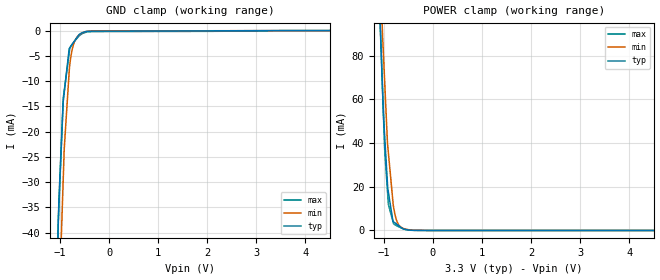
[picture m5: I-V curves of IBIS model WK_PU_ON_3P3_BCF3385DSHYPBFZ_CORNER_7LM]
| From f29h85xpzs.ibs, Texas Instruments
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|RECEIVER_MODE_3P3; RECEIVER_MODE
|   Model Cell WK_PU_ON_3P3_BCF3385DSHYPBFZ_CORNER_7LM
|WK_PU_ON_3P3_BCF3385DSHYPBFZ_CORNER_7LM
[Model]   WK_PU_ON_3P3_BCF3385DSHYPBFZ_CORNER_7LM
Model_type   Input
Polarity   Non-Inverting
Vinl = 0.8
Vinh = 2
|   typ   min   max
C_comp   0.44pF   0.4pF   0.46pF
[Model Spec]
Vinl   0.8   0.8   0.8
Vinh   2   2   2
[Temperature Range]   25   155   -40
[Voltage Range]   3.3   2.8   3.63
| Nom Voltages:
|   VDD=1.23, VDDS=3.3, VSS=0
| Min Voltages:
|   VDD=1.08, VDDS=2.8, VSS=0
| Max Voltages:
|   VDD=1.32, VDDS=3.63, VSS=0
[Power Clamp Reference]   3.3   2.8   3.63
[GND Clamp Reference]   0   0   0
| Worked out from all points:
|   GND clamp passes 1 mA (typ) near -0.63 V on its own axis
|   POWER clamp passes 1 mA (typ) near -0.63 V on its own axis
[GND Clamp]
|   Voltage   I(typ)   I(min)   I(max)
-3.3V     -1.475A    -1.211A    -2.162A
-1.048V   -42.98mA   -65.6mA    -41.49mA
-1.04V    -39.54mA   -62.41mA   -38.5mA
-1.024V   -33.55mA   -55.94mA   -34.71mA
-1.014V   -31.3mA    -52.41mA   -32.38mA
-939.6mV  -14.32mA   -30.43mA   -14.77mA
-933mV    -13.75mA   -28.47mA   -13.2mA
-915.9mV  -12.28mA   -23.41mA   -11.94mA
-809.2mV  -3.512mA   -7.267mA   -4.051mA
-718.9mV  -2.255mA   -2.517mA   -2.242mA
-550mV    -421.9uA   -464.8uA   -599.2uA
6.6V      0A         0A         0A
[POWER Clamp]
|   Voltage   I(typ)   I(min)   I(max)
-3.3V     1.946A     2.25A      2.109A
-1.079V   96.59mA    126.7mA    98.5mA
-1.036V   70.42mA    96.04mA    71.32mA
-1.004V   51.21mA    78.49mA    50.29mA
-979.5mV  41.85mA    66.43mA    35.68mA
-926.1mV  21.4mA     40.06mA    18.16mA
-907mV    17.44mA    35.44mA    11.89mA
-814.7mV  4.199mA    13.14mA    4.158mA
-784.9mV  3.688mA    8.638mA    2.783mA
-718.9mV  2.559mA    3.446mA    1.923mA
-615.8mV  793.7uA    1.094mA    900uA
6.6V      0A         0A         0A
